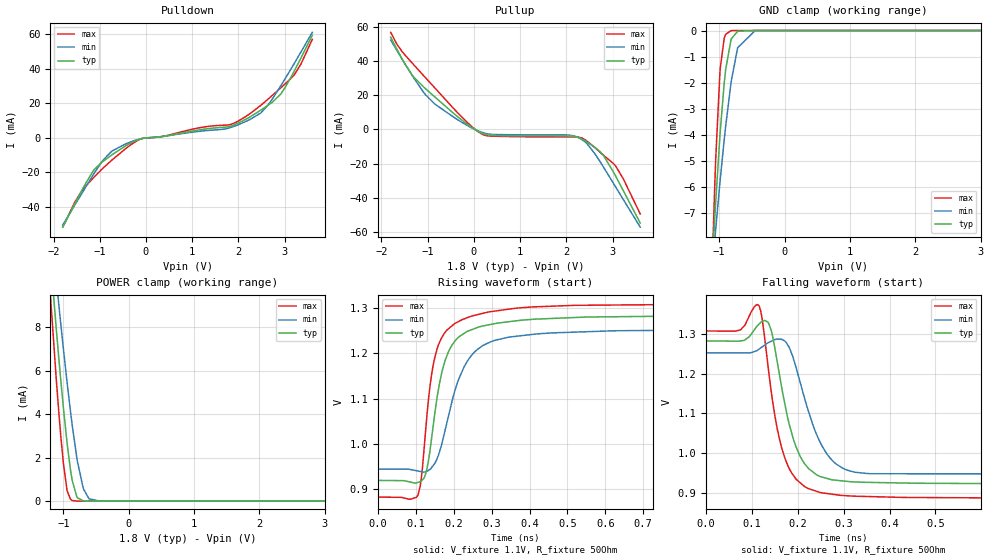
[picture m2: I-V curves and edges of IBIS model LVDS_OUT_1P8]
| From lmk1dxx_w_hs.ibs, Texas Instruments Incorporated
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|   LVDS_OUT_1P8 Model
[Model]   LVDS_OUT_1P8
Model_type   Output
Polarity   Non-Inverting
Vmeas = 1.1
Vref = 1.1
Cref = 2pF
Rref = 50
|   typ   min   max
C_comp   0.89pF   0.82pF   0.98pF
[Rac]   50   NA   NA
[Cac]   2p   NA   NA
[Voltage Range]   1.8   1.71   1.89
[Temperature Range]   45   150   -40
[Pullup Reference]   1.8   1.71   1.89
[Pulldown Reference]   -0   -0   -0
[Power Clamp Reference]   1.8   1.71   1.89
[GND Clamp Reference]   0   0   0
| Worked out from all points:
|   slope of the pulldown table from 0 to 0.27 V, typ, clamps not added: 523 ohm
|   slope of the pullup table from 0 to 0.27 V, typ, clamps not added: 78.5 ohm
|   GND clamp passes 1 mA (typ) near -0.87 V on its own axis
|   POWER clamp passes 1 mA (typ) near -0.87 V on its own axis
|   falling waveform, V_fixture 1.1V, R_fixture 50Ohm: 20-80 % time 46.8ps typ, 56.8ps min, 43.6ps max; typ from 1.28 V to 0.92 V
|   rising waveform, V_fixture 1.1V, R_fixture 50Ohm: 20-80 % time 51.6ps typ, 72.4ps min, 42.2ps max; typ from 0.92 V to 1.28 V
[Pulldown]
|   Voltage   I(typ)   I(min)   I(max)
-1.8V     -51.71mA   -50.47mA   -51.56mA
-1.531V   -37.8mA    -38.54mA   -36.82mA
-1.149V   -19.45mA   -21.75mA   -23.5mA
-918.7mV  -13.41mA   -12.59mA   -17.27mA
-735.7mV  -9.773mA   -7.629mA   -12.82mA
-87.12mV  -362uA     -378.6uA   -384.4uA
1.85V     6.976mA    6.159mA    7.951mA
2.488V    16.14mA    14.51mA    18.92mA
2.915V    25.34mA    30.07mA    28.95mA
3.21V     38.75mA    43.16mA    36.57mA
3.356V    46.4mA     49.88mA    42.9mA
3.6V      59.49mA    61.18mA    57.1mA
[GND Clamp]
|   Voltage   I(typ)   I(min)   I(max)
-1.8V     -47.22mA   -32.28mA   -90.43mA
-1.103V   -8.782mA   -9.069mA   -8.722mA
-1.072V   -7.372mA   -8.153mA   -6.225mA
-1.053V   -6.556mA   -7.61mA    -4.893mA
-988.9mV  -4.055mA   -5.855mA   -1.636mA
-982.4mV  -3.827mA   -5.684mA   -1.42mA
-922.5mV  -2.008mA   -4.177mA   -294.7uA
-899.8mV  -1.477mA   -3.648mA   -144.9uA
-818.3mV  -346uA     -1.998mA   -5.222uA
-717.3mV  -29.3uA    -659.5uA   -36.6nA
-450mV    -2.385nA   -3.724uA   -4.984pA
3.6V      0A         0A         0A
[Pullup]
|   Voltage   I(typ)   I(min)   I(max)
-1.8V     53.75mA    52.11mA    56.61mA
-1.668V   46.9mA     46.11mA    49.8mA
-1.327V   31.38mA    31.06mA    38.45mA
-1.045V   23.66mA    20.1mA     30.03mA
-450mV    9.556mA    7.303mA    12.45mA
163.4mV   -2.187mA   -1.661mA   -2.639mA
2.08V     -3.921mA   -3.483mA   -4.447mA
2.395V    -6.459mA   -7.117mA   -5.917mA
2.731V    -13.07mA   -18.89mA   -13.42mA
3.066V    -27.27mA   -33.63mA   -21.37mA
3.232V    -35.77mA   -40.93mA   -28.85mA
3.6V      -54.74mA   -57.17mA   -49.47mA
[POWER Clamp]
|   Voltage   I(typ)   I(min)   I(max)
-1.8V     35.35mA    33.02mA    38.41mA
-1.235V   12.58mA    14.14mA    11.07mA
-1.108V   7.901mA    10.18mA    5.58mA
-1.068V   6.535mA    8.999mA    4.045mA
-1V       4.324mA    7.032mA    1.764mA
-945.7mV  2.747mA    5.536mA    547.3uA
-890.1mV  1.424mA    4.11mA     81.35uA
-863.6mV  938uA      3.477mA    28.21uA
-793.4mV  199.1uA    1.989mA    1.463uA
-694.6mV  11.18uA    577.1uA    13.82nA
-607.7mV  708.9nA    109.9uA    193pA
3.6V      0A         0A         0A
[Ramp]
R_load = 50
|   typ   min   max
dV/dt_r   0.217774/5.15345e-11   0.184607/7.2296e-11   0.254891/4.20134e-11
dV/dt_f   0.218036/4.6756e-11   0.185102/5.68169e-11   0.254968/4.36722e-11
[Falling Waveform]
V_fixture = 1.1V
V_fixture_min = 1.1V
V_fixture_max = 1.1V
R_fixture = 50Ohm
C_fixture = 0F
|   Time   V(typ)   V(min)   V(max)
0s        1.283V     1.253V     1.308V
75.02ps   1.283V     1.253V     1.311V
115ps     1.325V     1.262V     1.373V
142.3ps   1.308V     1.282V     1.154V
156.1ps   1.223V     1.288V     1.056V
178.3ps   1.087V     1.272V     968mV
223.5ps   960.5mV    1.104V     910mV
252.6ps   939.4mV    1.018V     899.5mV
293.1ps   930.1mV    965.3mV    893.2mV
5ns       919.5mV    944.2mV    883.1mV
[Rising Waveform]
V_fixture = 1.1V
V_fixture_min = 1.1V
V_fixture_max = 1.1V
R_fixture = 50Ohm
C_fixture = 0F
|   Time   V(typ)   V(min)   V(max)
0s        919.8mV    945mV      883.1mV
105ps     915.4mV    940.6mV    886.9mV
115ps     919.3mV    939mV      932.4mV
125.1ps   934mV      939mV      1.028V
141.8ps   1.017V     948.9mV    1.157V
174.7ps   1.179V     1.023V     1.244V
209.6ps   1.234V     1.136V     1.269V
238.4ps   1.25V      1.187V     1.28V
362.6ps   1.272V     1.238V     1.3V
5ns       1.283V     1.253V     1.308V
